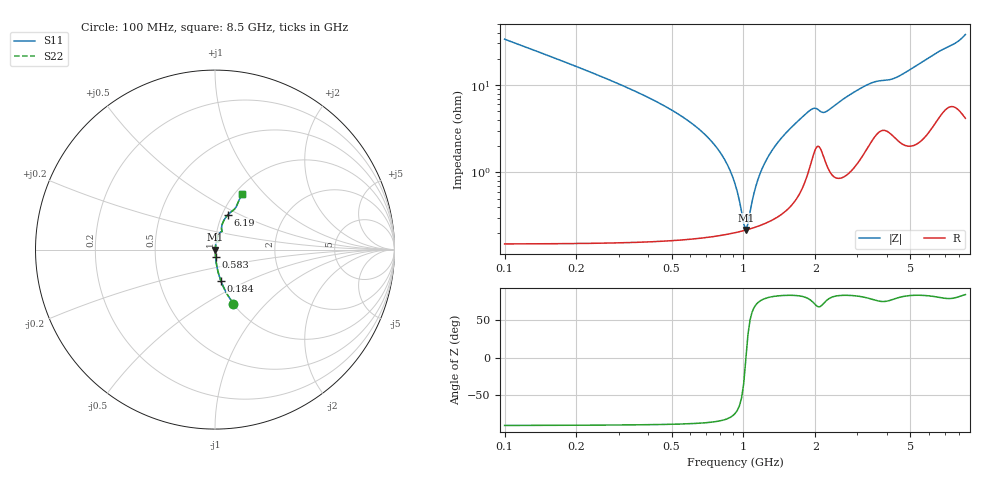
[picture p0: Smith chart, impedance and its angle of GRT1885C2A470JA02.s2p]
!Murata Part Number: GRT1885C2A470JA02
!These Parameters are Measured in Series Mode Connection
!Data Generated on Jun 19, 2026
!  o--ll--o
!Port1  Port2
!  o------o
!Operation Temp=25[degC], DC Bias Voltage=0[V]
!Freq. Start=100[MHz] Stop=9[GHz] 401[Steps]
# Hz S RI R 50
!Freq.(Hz) S11(Real) S11(Imag) S21(Real) S21(Imag) S12(Real) S12(Imag) S22(Real) S22(Imag)
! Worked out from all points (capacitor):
!   401 points, 100 MHz to 8.5 GHz, reference 50 ohm
!   read as one part in series: C = 47 pF near 142 MHz
!   lowest |Z| = 219 mohm at 1.024 GHz (marker M1)
!   series resonance near 1.025 GHz, so ESL is about 510 pH
!   S11 on the Smith chart (normalised r, x): 100 MHz: 1.00, -0.67; 184 MHz: 1.00, -0.36; 583 MHz: 1.00, -0.08; 6.19 GHz: 1.07, +0.43; 8.5 GHz: 1.08, +0.76
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1e8  0.1022 -0.3007  0.8978 0.3007  0.8978 0.3007  0.1022 -0.3007
1.84e8  0.0322 -0.1722  0.9678 0.1722  0.9678 0.1722  0.0322 -0.1722
3.31e8  0.00989 -0.0908  0.9901 0.0908  0.9901 0.0908  0.00989 -0.0908
5.83e8  0.00326 -0.0394  0.9967 0.0394  0.9967 0.0394  0.00326 -0.0394
8.35e8  0.00212 -0.0138  0.9979 0.0138  0.9979 0.0138  0.00212 -0.0138
9.19e8  0.00208 -0.00731  0.9979 0.00731  0.9979 0.00731  0.00208 -0.00731
9.82e8  0.00212 -0.00286  0.9979 0.00286  0.9979 0.00286  0.00212 -0.00286
1.024e9  0.00218 -3.49e-05  0.9978 3.49e-05  0.9978 3.49e-05  0.00218 -3.49e-05
1.045e9  0.00222 0.00134  0.9978 -0.00134  0.9978 -0.00134  0.00222 0.00134
1.129e9  0.00241 0.00661  0.9976 -0.00661  0.9976 -0.00661  0.00241 0.00661
1.213e9  0.00268 0.0116  0.9973 -0.0116  0.9973 -0.0116  0.00268 0.0116
1.339e9  0.00325 0.0187  0.9968 -0.0187  0.9968 -0.0187  0.00325 0.0187
1.507e9  0.00439 0.0278  0.9956 -0.0278  0.9956 -0.0278  0.00439 0.0278
1.927e9  0.0157 0.0496  0.9843 -0.0496  0.9843 -0.0496  0.0157 0.0496
2.2e9  0.0154 0.0459  0.9846 -0.0459  0.9846 -0.0459  0.0154 0.0459
2.914e9  0.0178 0.0803  0.9822 -0.0803  0.9822 -0.0803  0.0178 0.0803
3.481e9  0.0333 0.0987  0.9667 -0.0987  0.9667 -0.0987  0.0333 0.0987
4.3e9  0.037 0.1105  0.963 -0.1105  0.963 -0.1105  0.037 0.1105
5.707e9  0.0562 0.1738  0.9438 -0.1738  0.9438 -0.1738  0.0562 0.1738
6.19e9  0.0726 0.1945  0.9274 -0.1945  0.9274 -0.1945  0.0726 0.1945
7.114e9  0.1075 0.2243  0.8925 -0.2243  0.8925 -0.2243  0.1075 0.2243
8.5e9  0.1515 0.3076  0.8485 -0.3076  0.8485 -0.3076  0.1515 0.3076
